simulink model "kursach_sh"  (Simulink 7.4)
settings: Solver=ode45  StartTime=0.0  StopTime=8  RelTol=1e-3
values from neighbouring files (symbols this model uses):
  b1 = B(rezh,1)    [fash.m]    (also in kursach_ap_kren.m)
  b3 = B(rezh,3)    [fash.m]    (also in kursach_ap_kren.m)
undefined symbols (not defined in the file or in its folder): ie, myue, nyue

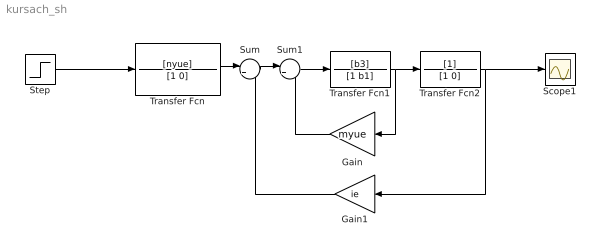
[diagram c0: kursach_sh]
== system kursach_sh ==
  Gain : Gain  Gain=myue  ParameterDataType=fixdt(1, 16)  ParameterScaling=2^0  OutDataType=fixdt(1, 16)  OutScaling=2^0
  Gain1 : Gain  Gain=ie  ParameterDataType=fixdt(1, 16)  ParameterScaling=2^0  OutDataType=fixdt(1, 16)  OutScaling=2^0
  Scope1 : Scope
  Step : Step  Time=2  Before=1  After=0  SampleTime=0
  Sum : Sum  Inputs=|+-  OutDataType=fixdt(1, 16)  OutScaling=2^0
  Sum1 : Sum  Inputs=|+-  OutDataType=fixdt(1, 16)  OutScaling=2^0
  Transfer Fcn : TransferFcn  Numerator=[nyue]  Denominator=[1 0]
  Transfer Fcn1 : TransferFcn  Numerator=[b3]  Denominator=[1 b1]
  Transfer Fcn2 : TransferFcn  Denominator=[1 0]
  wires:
  Transfer Fcn/1 -> Sum/1
  Sum/1 -> Sum1/1
  Sum1/1 -> Transfer Fcn1/1
  Gain/1 -> Sum1/2
  Transfer Fcn1/1 -> Transfer Fcn2/1, Gain/1
  Transfer Fcn2/1 -> Gain1/1, Scope1/1
  Gain1/1 -> Sum/2
  Step/1 -> Transfer Fcn/1
